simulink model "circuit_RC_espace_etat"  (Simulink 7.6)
settings: Solver=ode45  StartTime=0.0  StopTime=0.04  RelTol=1e-3
InitFcn:
  | R=2;
  | C=1e-3;
StopFcn:
  | load Vc_I_Creneau.mat
  | plot(x(1,:),x(2,:),x(1,:),x(3,:),x(1,:),x(4,:))
  | axis([0 0.04 -60 120])
  | grid
  | title('tension Vc, courant I et créneau d''entrée')
  | xlabel('temps')

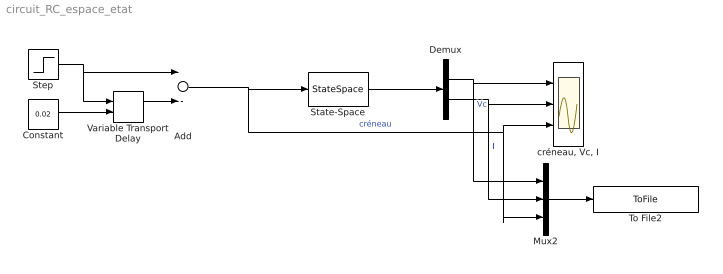
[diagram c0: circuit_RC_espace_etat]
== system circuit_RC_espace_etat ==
  Add : Sum  Inputs=+-
  Constant : Constant  Value=0.02
  Demux : Demux  Outputs=2
  Mux2 : Mux  Inputs=3
  State-Space : StateSpace  A=-1/(R*C)  B=1/(R*C)  C=[1 -1/R]'  D=[0 1/R]'
  Step : Step  Time=0.005  After=100  SampleTime=0
  To File2 : ToFile  Filename=Vc_I_Creneau  MatrixName=x
  Variable Transport Delay : VariableTransportDelay  VariableDelayType=Variable transport delay  MaximumDelay=10
  "créneau, Vc, I" : Scope  NumInputPorts=3
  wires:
  Add/1 -> State-Space/1, "créneau, Vc, I"/3, Mux2/3  "créneau"
  Step/1 -> Add/1, Variable Transport Delay/1
  Variable Transport Delay/1 -> Add/2
  Constant/1 -> Variable Transport Delay/2
  Demux/1 -> "créneau, Vc, I"/1, Mux2/1  "Vc"
  Demux/2 -> "créneau, Vc, I"/2, Mux2/2  "I"
  State-Space/1 -> Demux/1
  Mux2/1 -> To File2/1
